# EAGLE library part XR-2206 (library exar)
Monolithic FUNCTION GENERATOR
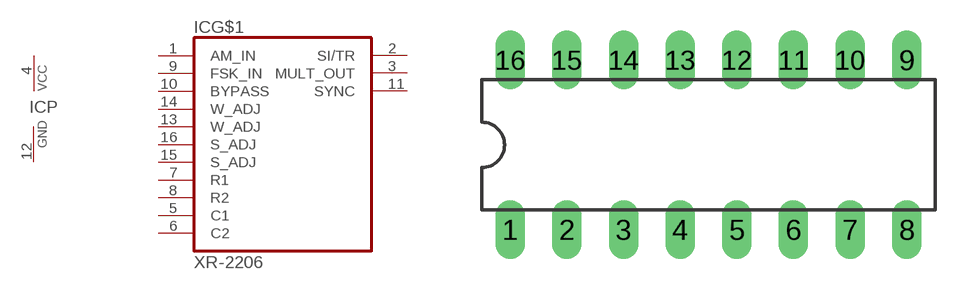
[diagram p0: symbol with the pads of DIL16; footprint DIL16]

Designator prefix IC; gates G$1=XR-2206 P=PWRN

## XR-2206 (OC_FARNELL: unknown; OC_NEWARK: unknown)  [DIL16]
1  G$1:AM_IN  in
2  G$1:SI/TR  out
3  G$1:MULT_OUT  out
4  P:VCC  pwr
5  G$1:C1  in
6  G$1:C2  in
7  G$1:R1  in
8  G$1:R2  in
9  G$1:FSK_IN  in
10  G$1:BYPASS  in
11  G$1:SYNC  out
12  P:GND  pwr
13  G$1:W_ADJ  in
14  G$1:W_ADJ  in
15  G$1:S_ADJ  in
16  G$1:S_ADJ  in

## Footprint DIL16 (pad centres in mm)
Dual In Line Package
drill 0.813 long: 1 -8.89,-3.81; 2 -6.35,-3.81; 3 -3.81,-3.81; 4 -1.27,-3.81; 5 1.27,-3.81; 6 3.81,-3.81; 7 6.35,-3.81; 8 8.89,-3.81; 9 8.89,3.81; 10 6.35,3.81; 11 3.81,3.81; 12 1.27,3.81; 13 -1.27,3.81; 14 -3.81,3.81; 15 -6.35,3.81; 16 -8.89,3.81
